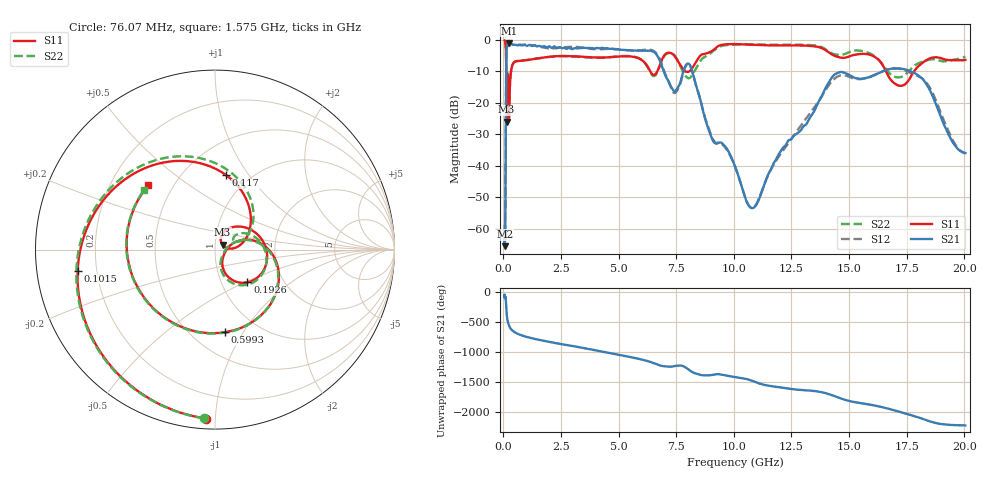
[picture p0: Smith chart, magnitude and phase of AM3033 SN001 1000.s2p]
# Hz S DB R 50
!freq MagS11 AngS11 MagS21 AngS21 MagS12 AngS12 MagS22 AngS22
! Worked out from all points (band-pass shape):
!   1601 points, 50 MHz to 20.05 GHz, reference 50 ohm
!   highest |S21| = -0.94 dB at 257 MHz (marker M1); lowest = -65.6 dB at 54.09 MHz (marker M2)
!   |S21| within 3 dB of the highest: 128.4 MHz to 6.571 GHz (6.443 GHz wide, 192 % of centre)
!   lowest |S11| = -25.9 dB at 133.4 MHz (marker M3), VSWR 1.11, Z = 54.3 + j3.08 ohm
!   |S11| at or under -10 dB: 120.1 MHz to 327.2 MHz (207.1 MHz wide, 92.6 % of centre); 6.376 GHz to 6.673 GHz (297.1 MHz wide, 4.55 % of centre); 16.6 GHz to 17.82 GHz (1.217 GHz wide, 7.07 % of centre)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
!   |S22| runs from -25.8 to -0.1 dB; largest |S21 - S12| = 0.063
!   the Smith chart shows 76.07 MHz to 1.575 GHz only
!   S11 on the Smith chart (normalised r, x): 76.07 MHz: 0.06, -0.95; 101.5 MHz: 0.13, -0.07; 117 MHz: 0.78, +0.79; 192.6 MHz: 1.32, -0.52; 599.3 MHz: 0.71, -0.83; 1.575 GHz: 0.37, +0.36
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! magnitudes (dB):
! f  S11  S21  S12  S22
! 50 MHz  -0.1  -61.7  -58.8  -0.1
! 54.09 MHz  -0.2  -65.6  -63.9  -0.2
! 76.07 MHz  -0.5  -61.8  -61.0  -0.5
! 101.5 MHz  -2.2  -28.5  -28.5  -2.2
! 117 MHz  -7.5  -9.2  -9.2  -7.0
! 133.4 MHz  -25.9  -3.2  -3.2  -18.8
! 135.9 MHz  -24.8  -3.0  -3.0  -18.5
! 155 MHz  -12.3  -2.3  -2.2  -11.9
! 192.6 MHz  -11.8  -1.5  -1.6  -11.9
! 257 MHz  -20.3  -0.9  -0.9  -20.3
! 369.6 MHz  -8.4  -1.4  -1.3  -8.4
! 599.3 MHz  -6.7  -1.6  -1.5  -6.6
! 1.005 GHz  -6.4  -1.8  -1.5  -6.4
! 1.575 GHz  -5.8  -1.9  -2.1  -5.8
! 2.722 GHz  -5.1  -2.8  -2.4  -5.1
! 6.396 GHz  -10.3  -3.4  -3.1  -10.5
! 7.402 GHz  -4.9  -16.2  -16.8  -4.6
! 8.129 GHz  -9.6  -8.4  -8.7  -11.8
! 10.77 GHz  -1.5  -53.5  -53.3  -1.4
! 14.58 GHz  -5.5  -10.2  -11.4  -4.7
! 17.78 GHz  -10.4  -10.3  -10.8  -8.5
! 20.05 GHz  -6.3  -35.9  -36.1  -5.3
